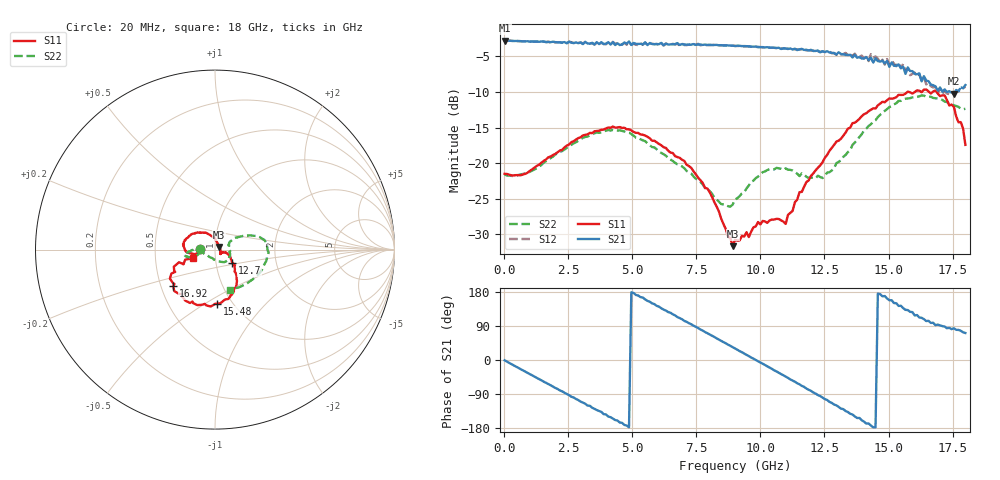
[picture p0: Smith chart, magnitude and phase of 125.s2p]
!Agilent Technologies,N5230A,US43500223,A.07.50.48
!Agilent N5230A: A.07.50.48
!Date: Sunday, January 10, 2016 21:01:03
!Correction: S11(Full 2 Port(1,2))
!S21(Full 2 Port(1,2))
!S12(Full 2 Port(1,2))
!S22(Full 2 Port(1,2))
!S2P File: Measurements: S11, S21, S12, S22:
# Hz S  dB  R 50
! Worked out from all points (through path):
!   201 points, 20 MHz to 18 GHz, reference 50 ohm
!   highest |S21| = -2.79 dB at 20 MHz (marker M1); lowest = -10.3 dB at 17.55 GHz (marker M2)
!   group delay of S21, straight-line fit = 103 ps
!   lowest |S11| = -31.6 dB at 8.92 GHz (marker M3), VSWR 1.05, Z = 52.2 + j1.48 ohm
!   |S11| at or under -10 dB: start of sweep to 15.74 GHz; 15.79 GHz to 16.03 GHz (234.1 MHz wide, 1.47 % of centre); 16.88 GHz to end of sweep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
!   |S22| runs from -26.1 to -10.5 dB; largest |S21 - S12| = 0.05
!   S11 on the Smith chart (normalised r, x): 20 MHz: 0.84, +0.00; 12.7 GHz: 1.20, -0.18; 15.48 GHz: 0.85, -0.56; 16.92 GHz: 0.58, -0.26; 18 GHz: 0.77, -0.08
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2e7  -21.50 179.2  -2.79 -0.8  -2.78 -0.8  -21.58 179.0
1.5483e9  -19.67 -167.5  -2.93 -57.4  -2.95 -57.6  -19.90 -163.2
2.3574e9  -17.77 -170.0  -3.01 -86.6  -3.00 -86.3  -18.08 -162.2
3.0766e9  -16.09 -174.3  -3.29 -112.5  -3.21 -112.5  -16.44 -163.1
4.0655e9  -14.99 173.5  -3.02 -149.2  -3.04 -148.3  -15.34 -167.9
4.8746e9  -15.24 159.8  -2.92 -177.6  -3.00 -177.1  -15.73 -172.9
6.0433e9  -17.30 135.4  -3.30 140.9  -3.42 141.3  -18.35 -179.2
6.7625e9  -19.14 121.0  -3.15 113.3  -3.24 112.9  -20.16 179.8
7.5716e9  -22.04 105.5  -3.34 84.4  -3.25 83.8  -22.38 -170.9
8.9201e9  -31.64 32.8  -3.50 33.7  -3.52 33.9  -25.80 -102.9
9.01e9  -30.75 17.5  -3.57 30.4  -3.54 30.5  -25.10 -97.8
1.04484e10  -27.91 -36.4  -3.78 -23.3  -3.79 -23.5  -20.91 -44.4
1.09878e10  -28.51 -22.6  -3.91 -43.9  -3.89 -43.9  -20.73 -27.8
1.20666e10  -21.43 -20.6  -4.26 -85.8  -4.21 -85.4  -22.02 7.3
1.26959e10  -18.27 -37.1  -4.46 -110.5  -4.32 -110.7  -21.27 24.9
1.43141e10  -12.50 -60.2  -5.21 -172.9  -4.71 -171.5  -14.54 24.2
1.50333e10  -10.90 -75.0  -6.48 157.7  -6.20 157.9  -12.11 17.1
1.54828e10  -10.42 -87.8  -6.67 143.2  -6.67 138.6  -11.25 12.0
1.6202e10  -9.84 -112.1  -7.39 112.1  -7.58 111.3  -10.61 -1.5
1.69212e10  -10.22 -138.9  -9.81 93.3  -10.19 93.3  -10.91 -22.7
1.75505e10  -12.09 -157.3  -10.26 83.8  -10.30 82.4  -11.88 -50.9
1.8e10  -17.43 -158.8  -9.03 71.2  -9.27 71.6  -12.37 -69.1
